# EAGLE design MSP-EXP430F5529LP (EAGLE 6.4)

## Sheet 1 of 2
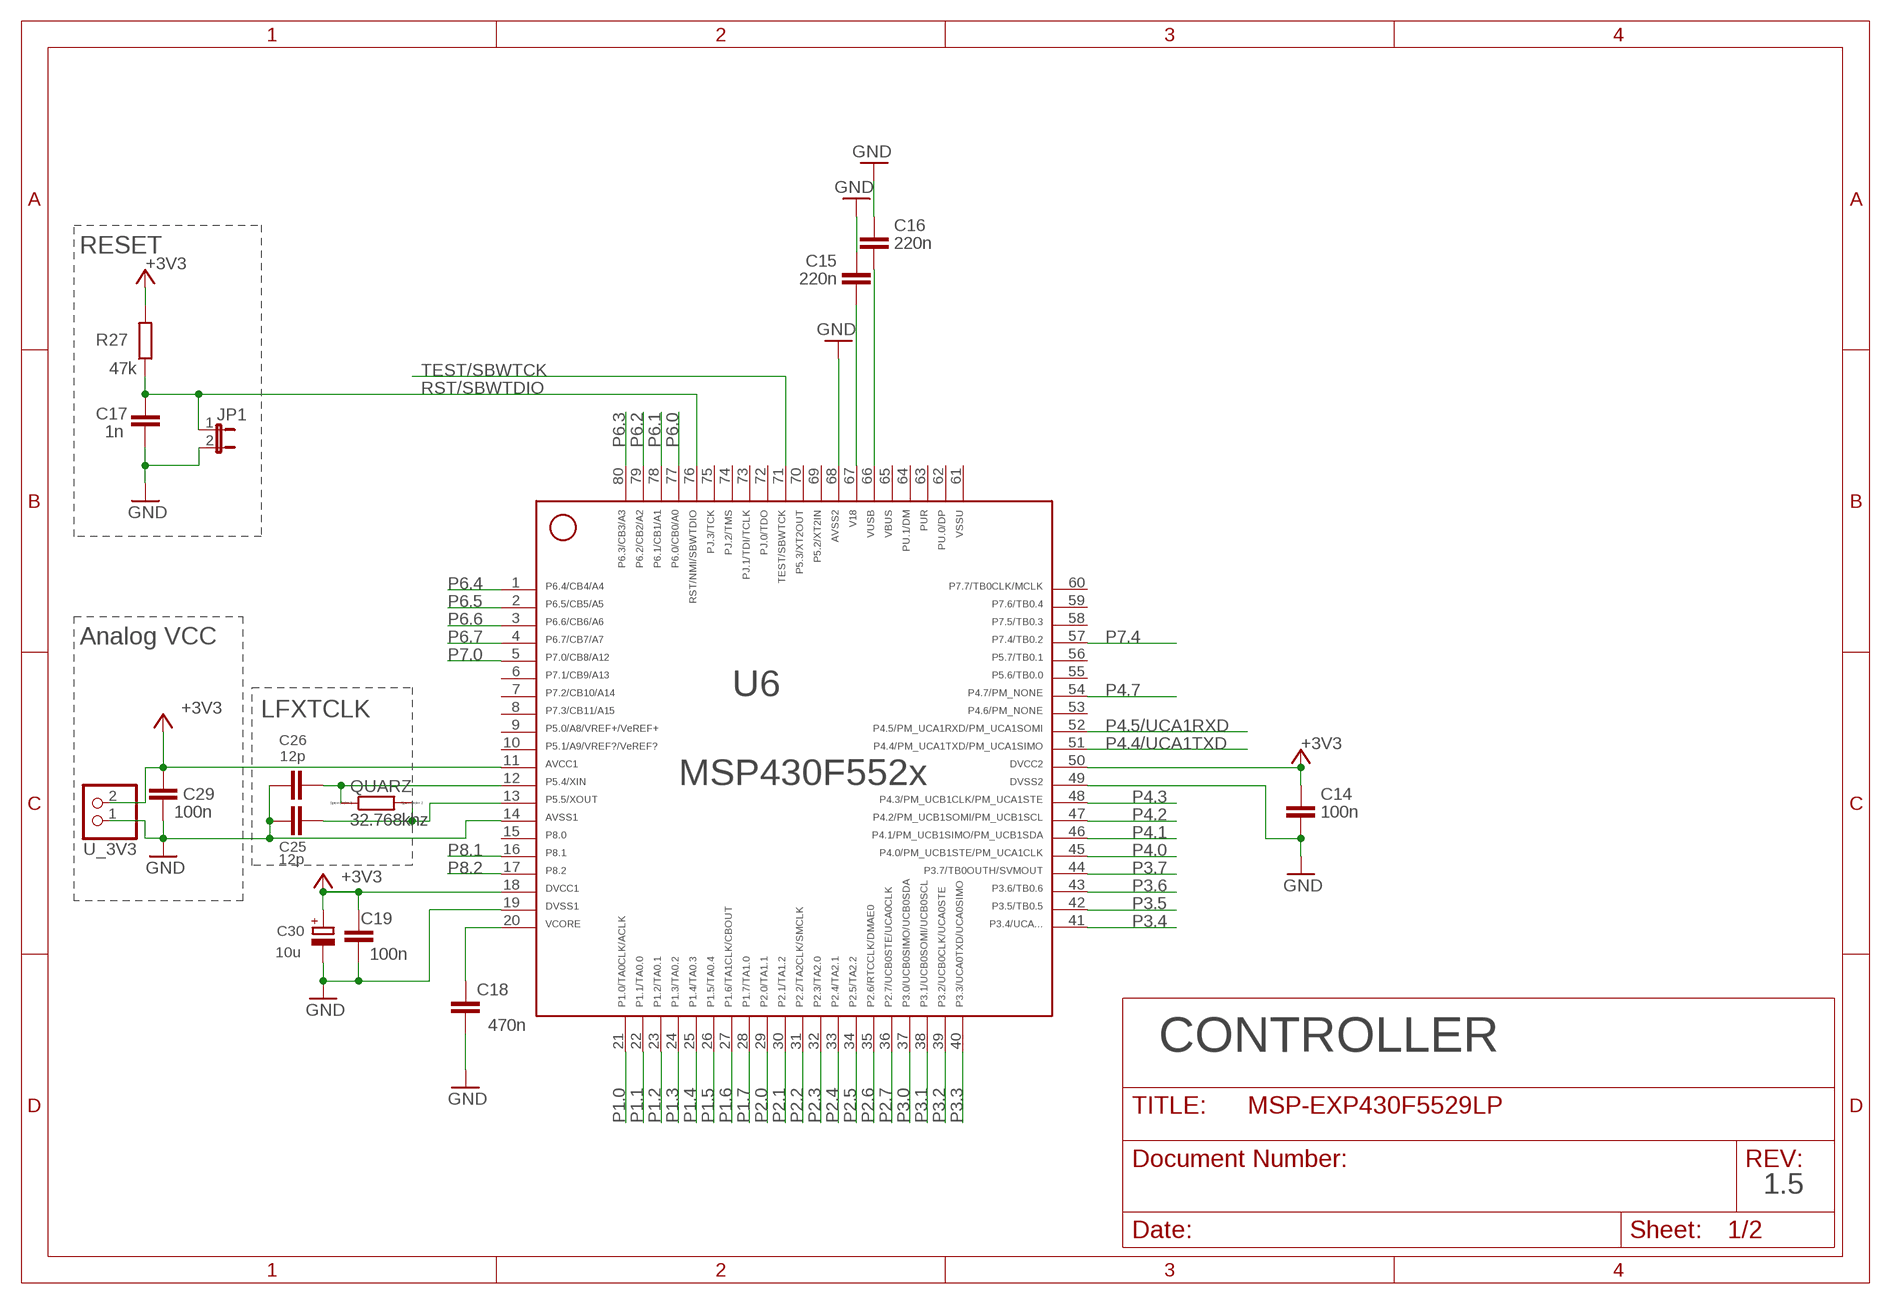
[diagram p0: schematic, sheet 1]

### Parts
C14  100n  C-EUC0402  [C0402]
C15  220n  C-EUC0805  [C0805]
C16  220n  C-EUC0805  [C0805]
C17  1n  C-EUC0805  [C0805]
C18  470n  C-EUC0805  [C0805]
C19  100n  C-EUC0603  [C0603]
C25  12p  C-EUC0805  [C0805]
C26  12p  C-EUC0805  [C0805]
C29  100n  C-EUC0603  [C0603]
C30  10u  CPOL-EUA/3216-18R  [A/3216-18R]
JP1  JP1E  [JP1]
QUARZ  32.768khz  RR1206  [R1206]
R27  47k  R-EU_R0603  [R0603]
U6  MSP430F5529IPNR  F552X---PN80  [PN80]
U_3V3  PINHD-1X2  [1X02]

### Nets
+3V3 [Power]: C14.1 C19.2 C29.1 C30.+ R27.2 U6.11 U6.18 U6.50 U_3V3.2 ; also sheet 2
GND [Ground]: C14.2 C15.2 C16.2 C17.2 C18.1 C19.1 C25.1 C26.1 C29.2 C30.- JP1.2 U6.14 U6.19 U6.49 U6.68 U_3V3.1 ; also sheet 2
P1.0: U6.21 ; also sheet 2
P1.1: U6.22
P1.2: U6.23 ; also sheet 2
P1.3: U6.24 ; also sheet 2
P1.4: U6.25 ; also sheet 2
P1.5: U6.26 ; also sheet 2
P1.6: U6.27 ; also sheet 2
P1.7: U6.28
P2.0: U6.29
P2.1: U6.30
P2.2: U6.31
P2.3: U6.32
P2.4: U6.33
P2.5: U6.34
P2.6: U6.35 ; also sheet 2
P2.7: U6.36
P3.0: U6.37 ; also sheet 2
P3.1: U6.38
P3.2: U6.39 ; also sheet 2
P3.3: U6.40 ; also sheet 2
P3.4: U6.41
P3.5: U6.42 ; also sheet 2
P3.6: U6.43 ; also sheet 2
P3.7: U6.44
P4.0: U6.45
P4.1: U6.46 ; also sheet 2
P4.2: U6.47
P4.3: U6.48 ; also sheet 2
P4.4/UCA1TXD: U6.51 ; also sheet 2
P4.5/UCA1RXD: U6.52 ; also sheet 2
P4.7: U6.54 ; also sheet 2
P5.4/XIN: C26.2 QUARZ.1 U6.12
P5.5/XOUT: C25.2 QUARZ.2 U6.13
P6.0: U6.77 ; also sheet 2
P6.1: U6.78 ; also sheet 2
P6.2: U6.79 ; also sheet 2
P6.3: U6.80 ; also sheet 2
P6.4: U6.1
P6.5: U6.2
P6.6: U6.3
P6.7: U6.4
P7.0: U6.5
P7.4: U6.57 ; also sheet 2
P8.1: U6.16 ; also sheet 2
P8.2: U6.17
RST/SBWTDIO: C17.1 JP1.1 R27.1 U6.76 ; also sheet 2
TARGET_VUSB [Power]: C16.1 U6.66
TEST/SBWTCK: U6.71 ; also sheet 2
V18 [Power]: C15.1 U6.67
VCORE [Power]: C18.2 U6.20
Unconnected: U6.6 U6.7 U6.8 U6.9 U6.10 U6.15 U6.53 U6.55 U6.56 U6.58 U6.59 U6.60 U6.62 U6.63 U6.64 U6.69 U6.70 U6.72 U6.73 U6.74 U6.75

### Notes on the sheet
- RESET
- Analog VCC
- LFXTCLK
- CONTROLLER
- 1.5

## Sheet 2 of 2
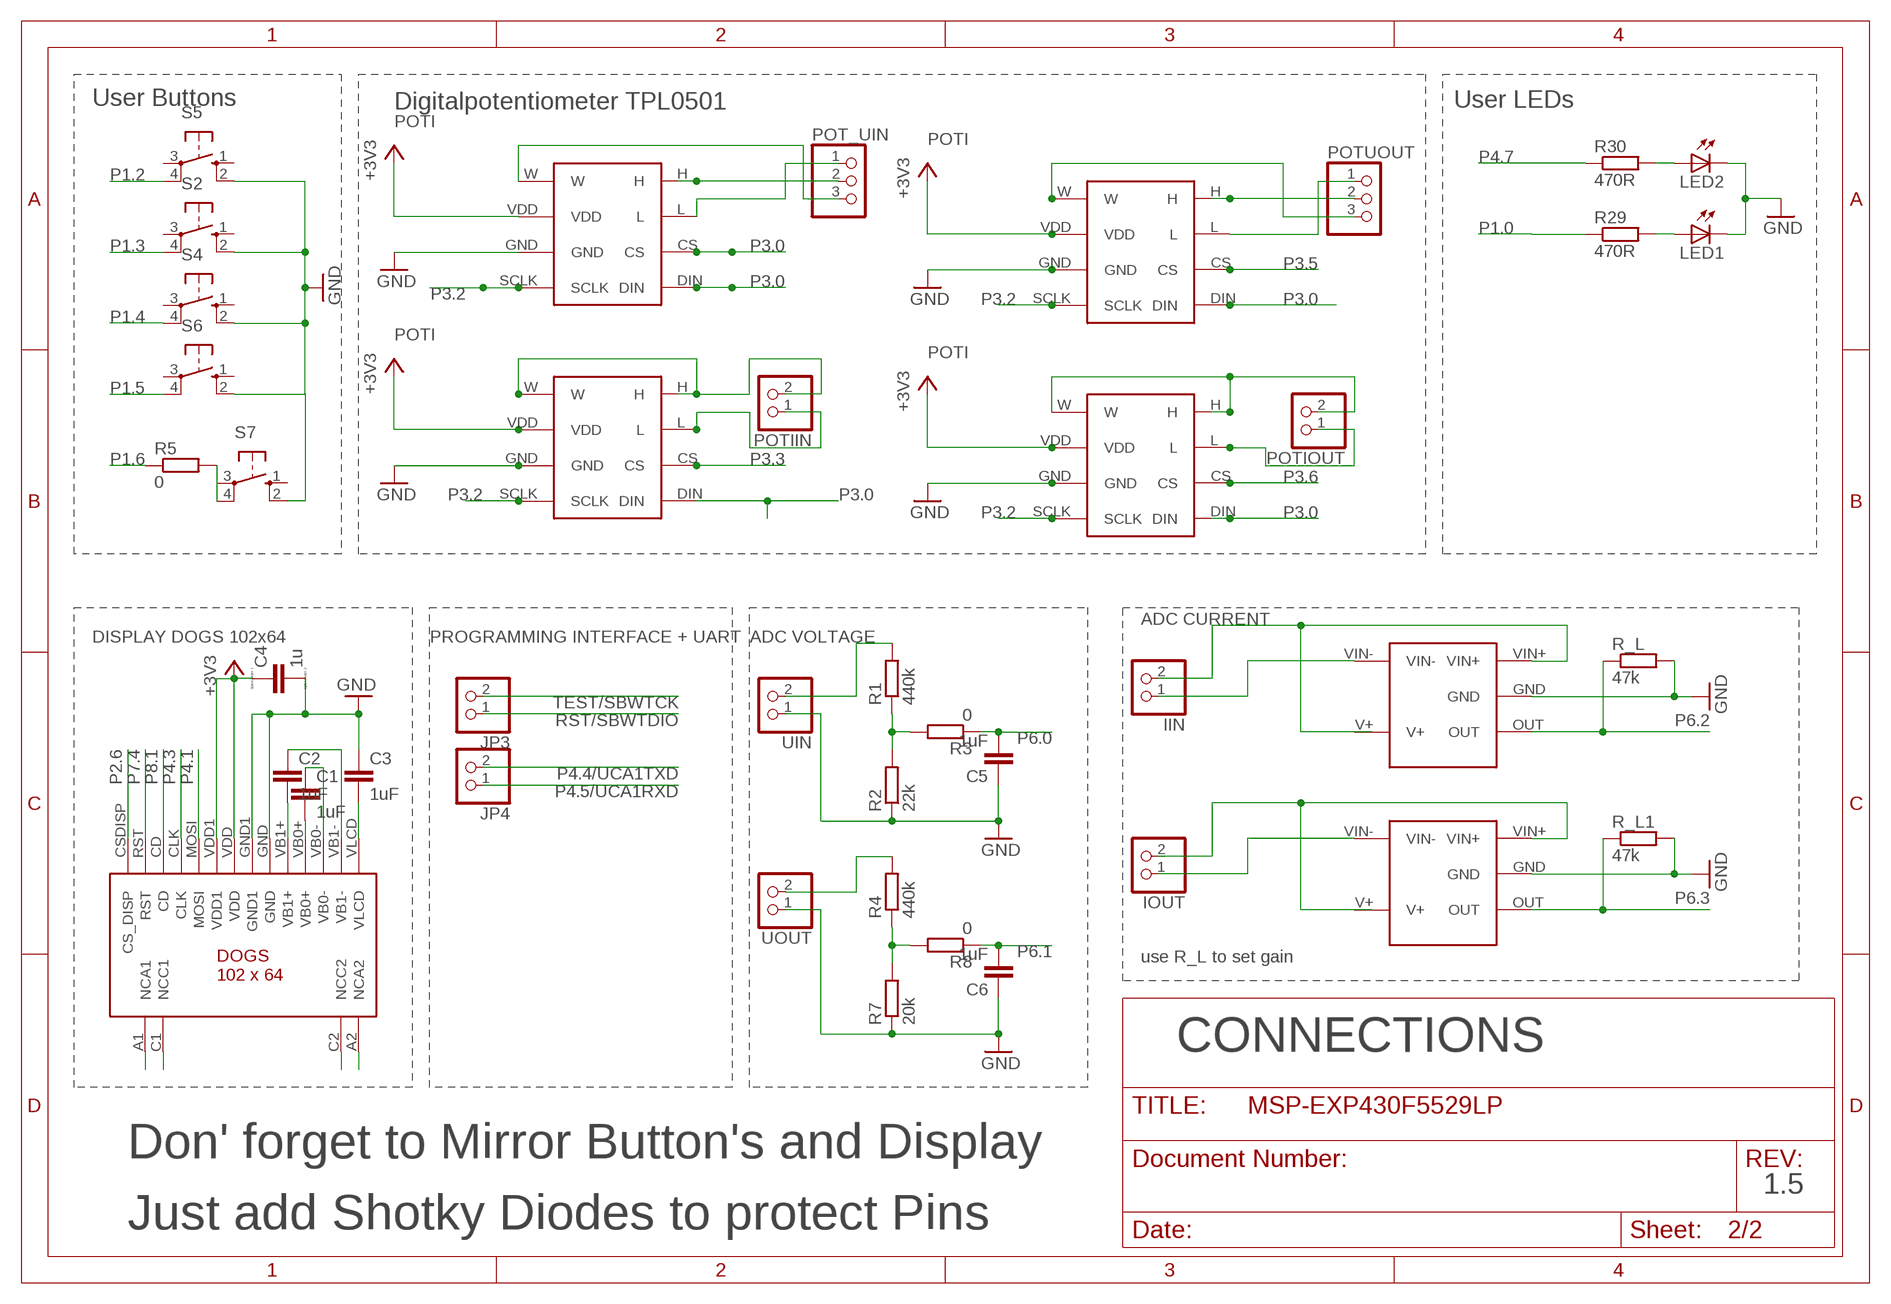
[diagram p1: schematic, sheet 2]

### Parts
C1  1uF  C-EUC0805  [C0805]
C2  1uF  C-EUC0805  [C0805]
C3  1uF  C-EUC0805  [C0805]
C4  1u  C  [C0805]
C5  1uF  C-EUC0805  [C0805]
C6  1uF  C-EUC0805  [C0805]
IIN  PINHD-1X2  [1X02]
IOUT  PINHD-1X2  [1X02]
JP3  PINHD-1X2  [1X02]
JP4  PINHD-1X2  [1X02]
LED1  LEDCHIP-LED0805  [CHIP-LED0805]
LED2  LEDCHIPLED_0603  [CHIPLED_0603]
POT_UIN  PINHD-1X3  [1X03]
POTIIN  PINHD-1X2  [1X02]
POTIOUT  PINHD-1X2  [1X02]
POTUOUT  PINHD-1X3  [1X03]
R1  440k  R-EU_MELF0204W  [MINI_MELF-0204W]
R2  22k  R-EU_R0805  [R0805]
R3  0  R-EU_R0805  [R0805]
R4  440k  R-EU_R0805  [R0805]
R5  0  R-EU_R0805  [R0805]
R7  20k  R-EU_R0805  [R0805]
R8  0  R-EU_R0805  [R0805]
R29  470R  R-EU_R0805  [R0805]
R30  470R  R-EU_R0603  [R0603]
R_L  47k  R-EU_M0805  [M0805]
R_L1  47k  R-EU_M0805  [M0805]
S2  10-XX  [B3F-10XX]
S4  10-XX  [B3F-10XX]
S5  10-XX  [B3F-10XX]
S6  10-XX  [B3F-10XX]
S7  10-XX  [B3F-10XX]
U$1  INA138  [SOT23-5]
U$2  INA138  [SOT23-5]
U$4  TPL0501  [SOT23-8L]
U$6  TPL0501  [SOT23-8L]
U$7  TPL0501  [SOT23-8L]
U$8  TPL0501  [SOT23-8L]
U$9  DOGS102  [1X14]
UIN  PINHD-1X2  [1X02]
UOUT  PINHD-1X2  [1X02]

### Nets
+3V3 [Power]: C4.1 U$4.VDD U$6.VDD U$7.VDD U$8.VDD U$9.VDD U$9.VDD1 ; also sheet 1
GND [Ground]: C3.1 C4.2 C5.1 C6.1 LED1.C LED2.C R2.1 R7.1 R_L1.2 R_L.2 S2.2(S1) S4.2(S1) S5.2(S1) S6.2(S1) S7.2(S1) U$1.GND U$2.GND U$4.GND U$6.GND U$7.GND U$8.GND U$9.GND U$9.GND1 UIN.1 UOUT.1 ; also sheet 1
N$1: POT_UIN.2 U$4.H
N$2: POTIIN.1 U$6.L
N$3: POT_UIN.1 U$4.L
N$4: POT_UIN.3 U$4.W
N$5: POTUOUT.3 U$8.W
N$6: IIN.2 U$1.VIN+
N$7: C2.2 U$9.VB1+
N$8: POTIOUT.1 U$7.L
N$9: R1.1 R2.2 R3.2
N$12: POTIIN.2 U$6.H U$6.W
N$13: POTUOUT.2 U$8.H
N$14: POTUOUT.1 U$8.L
N$15: R5.2 S7.4(P1)
N$16: C1.2 U$9.VB0+
N$17: C1.1 U$9.VB0-
N$18: C2.1 U$9.VB1-
N$19: C3.2 U$9.VLCD
N$22: U$9.A1(NCA1)
N$23: U$9.C1(NCC1)
N$24: IIN.1 U$1.VIN-
N$26: R1.2 UIN.2
N$28: U$9.C2(NCC2)
N$30: IOUT.2 U$2.VIN+
N$32: LED1.A R29.2
N$34: IOUT.1 U$2.VIN-
N$35: LED2.A R30.2
N$36: U$9.A2(NCA2)
N$37: R4.1 R7.2 R8.2
N$39: R4.2 UOUT.2
N$44: POTIOUT.2 U$7.H U$7.W
P1.0: R29.1 ; also sheet 1
P1.2: S5.4(P1) ; also sheet 1
P1.3: S2.4(P1) ; also sheet 1
P1.4: S4.4(P1) ; also sheet 1
P1.5: S6.4(P1) ; also sheet 1
P1.6: R5.1 ; also sheet 1
P2.6: U$9.CSDISP(CS_DISP) ; also sheet 1
P3.0: U$4.CS U$4.DIN U$6.DIN U$7.DIN U$8.DIN ; also sheet 1
P3.2: U$4.SCLK U$6.SCLK U$7.SCLK U$8.SCLK ; also sheet 1
P3.3: U$6.CS ; also sheet 1
P3.5: U$8.CS ; also sheet 1
P3.6: U$7.CS ; also sheet 1
P4.1: U$9.MOSI ; also sheet 1
P4.3: U$9.CLK ; also sheet 1
P4.4/UCA1TXD: JP4.2 ; also sheet 1
P4.5/UCA1RXD: JP4.1 ; also sheet 1
P4.7: R30.1 ; also sheet 1
P6.0: C5.2 R3.1 ; also sheet 1
P6.1: C6.2 R8.1 ; also sheet 1
P6.2: R_L.1 U$1.OUT ; also sheet 1
P6.3: R_L1.1 U$2.OUT ; also sheet 1
P7.4: U$9.RST ; also sheet 1
P8.1: U$9.CD ; also sheet 1
RST/SBWTDIO: JP3.1 ; also sheet 1
TEST/SBWTCK: JP3.2 ; also sheet 1
Unconnected: S2.1(S) S2.3(P) S4.1(S) S4.3(P) S5.1(S) S5.3(P) S6.1(S) S6.3(P) S7.1(S) S7.3(P) U$1.V+ U$2.V+

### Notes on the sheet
- User Buttons | Digitalpotentiometer TPL0501 | User LEDs
- POTI
- POTI
- POTI
- POTI
- ADC CURRENT
- DISPLAY DOGS 102x64 | PROGRAMMING INTERFACE + UART | ADC VOLTAGE
- use R_L to set gain
- CONNECTIONS
- Don' forget to Mirror Button's and Display
- 1.5
- Just add Shotky Diodes to protect Pins

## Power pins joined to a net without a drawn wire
61: U6.61
65: U6.65

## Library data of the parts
C1-C3 C5 C6 C14-C19 C25 C26 C29 = rcl:C-EU: CAPACITOR, European symbol
C4 = eagle-ltspice:C: CAPACITOR, European symbol; SPICEMODEL: NONE; SPICEPREFIX: C
C30 = rcl:CPOL-EU: POLARIZED CAPACITOR, European symbol
IIN IOUT JP3 JP4 POTIIN POTIOUT U_3V3 UIN UOUT = pinhead:PINHD-1X2: PIN HEADER
JP1 = jumper:JP1E: JUMPER
LED1 LED2 = led:LED: LED
POT_UIN POTUOUT = pinhead:PINHD-1X3: PIN HEADER
QUARZ = eagle-ltspice:R: RESISTOR, European symbol; SPICEMODEL: NONE; SPICEPREFIX: R
R1-R5 R7 R8 R27 R29 R30 R_L R_L1 = rcl:R-EU_: RESISTOR, European symbol
S2 S4-S7 = switch-omron:10-XX: OMRON SWITCH; MPN: B3F-1000; OC_FARNELL: 176432; OC_NEWARK: 36M3542
U6 = TI_MSP430_v16_intern:F552X---PN80: ***MSP430F552X***PN80 http://www.ti.com/lit/gpn/msp430f5529 Rev1.0 06/2010 For F552X where X is 1,5,7,9
U$1 U$2 = current_shunt:INA138
U$4 U$6-U$8 = tpl0501:TPL0501
U$9 = dogs_102x64:DOGS102

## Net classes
0 Default: width 0.203 mm, drill 0.305 mm, clearance 0.152 mm
1 Ground: width 0.203 mm, drill 0.305 mm, clearance 0.152 mm to class 0, clearance 0.152 mm
2 Power: width 0.203 mm, drill 0.305 mm, clearance 0.152 mm to class 0, clearance 0.152 mm to class 1, clearance 0.152 mm

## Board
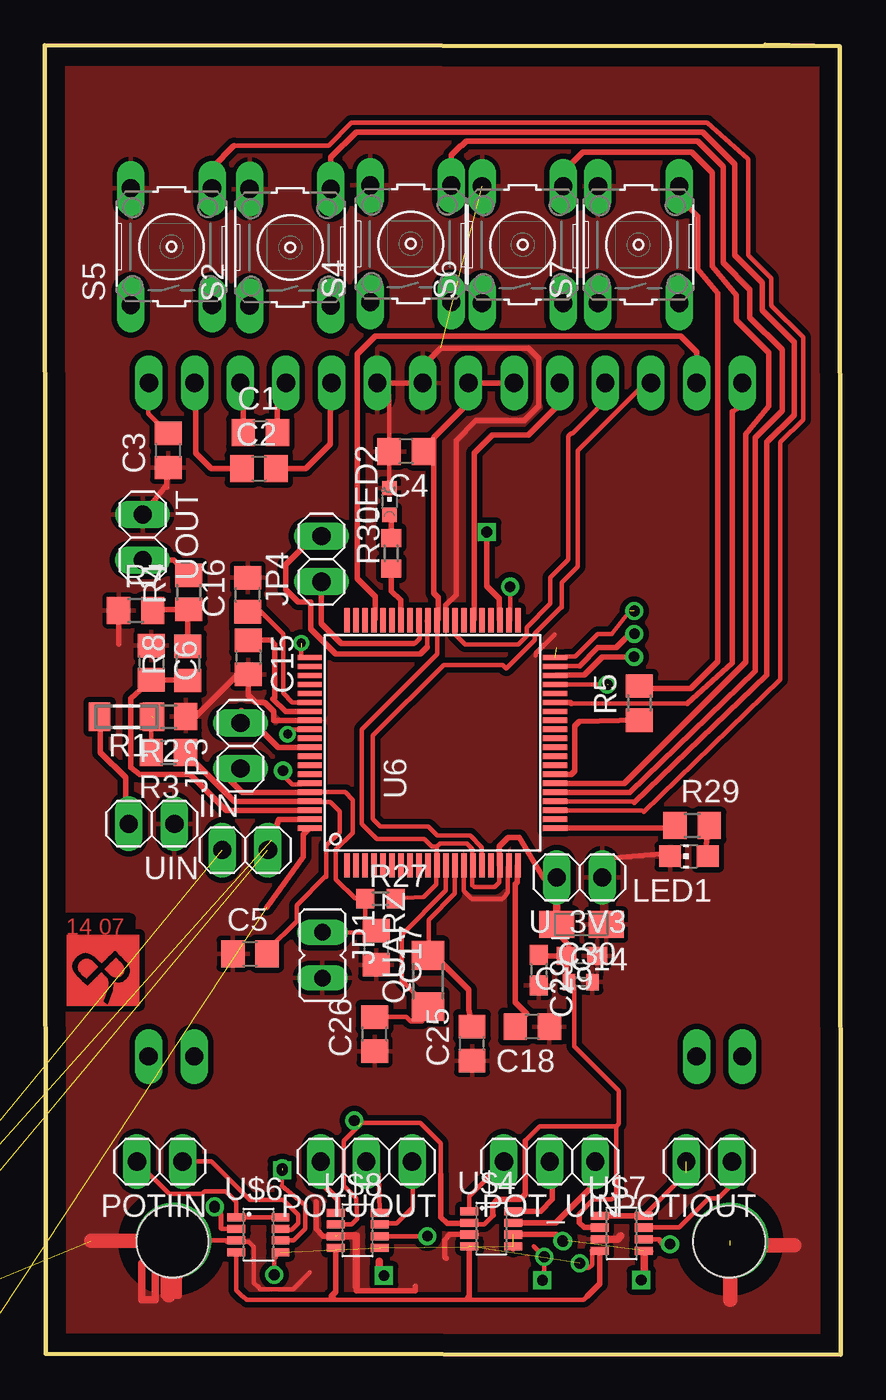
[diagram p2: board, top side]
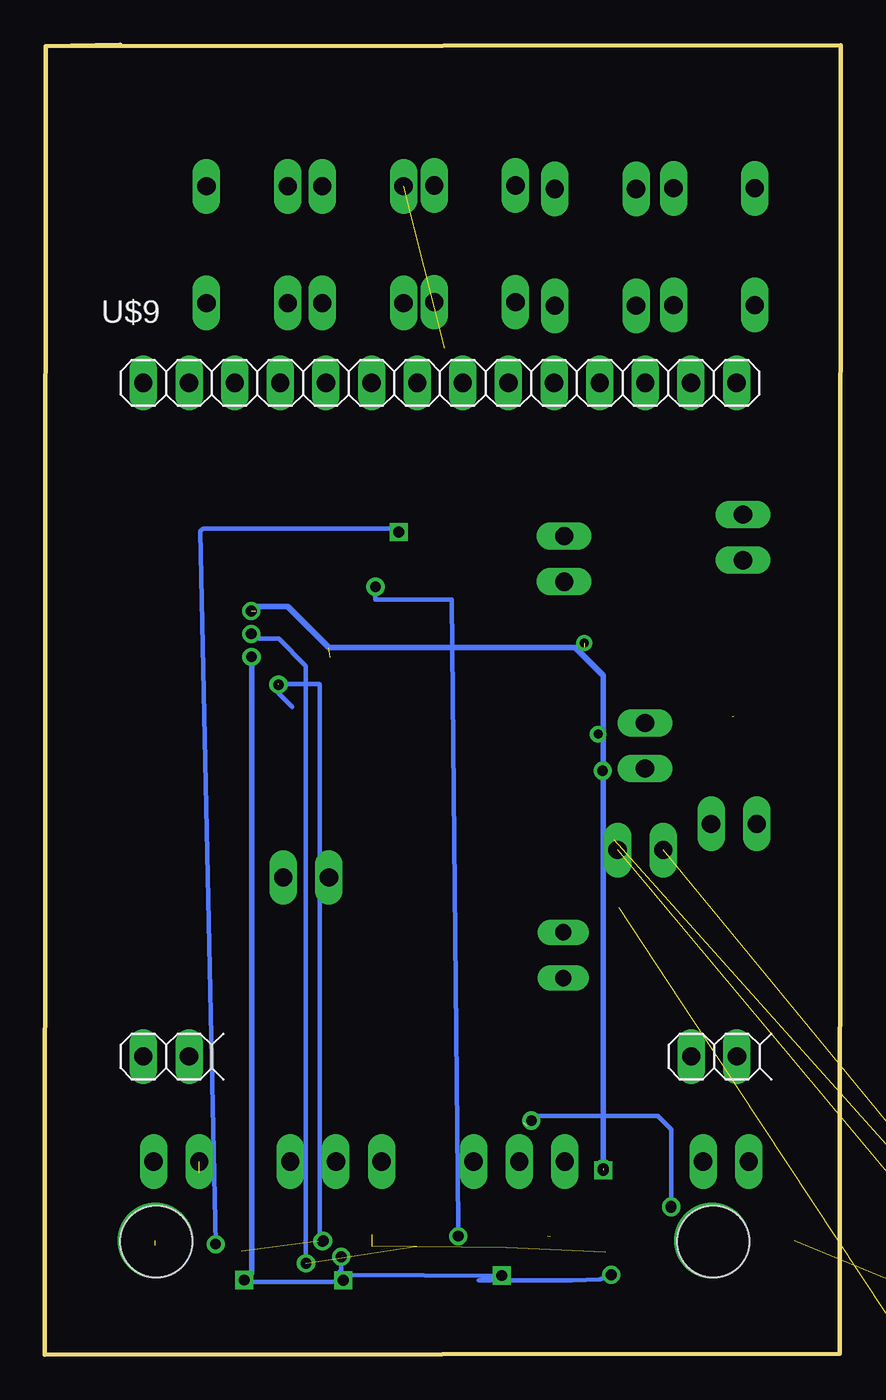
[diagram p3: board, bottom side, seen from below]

Size 44.29 x 72.92 mm. Coordinates in mm from the lower left corner, seen from the top.
Outline: 40.09,72.92 44.25,72.84
Outline: 44.25,72.84 44.29,0 0.04,0.05 0,72.89 44.25,72.84
Copper layers (1*16): Top 0.035mm / dielectric 1.5mm / Bottom 0.035mm
Design rules "default": minimum track width 10mil, minimum drill 24mil, track to track 8mil, track to pad 8mil, pad to pad 8mil, via to via 8mil, smd to smd 8mil, copper to edge 40mil, drill to drill 8mil, minimum pad ring 10mil, minimum via ring 8mil, stop-mask expansion 4mil, vias tented up to drill 0mil, thermal gap 10mil
Holes 4 mm at 7.09,6.3 38.09,6.3

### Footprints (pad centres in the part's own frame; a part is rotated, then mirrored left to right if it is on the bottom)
C0805 = smd 1.3 x 1.5: 1 -0.95,0; 2 0.95,0
C0402 = smd 0.7 x 0.9: 1 -0.65,0; 2 0.65,0
C0603 = smd 1.1 x 1: 1 -0.85,0; 2 0.85,0
A/3216-18R = smd 1.95 x 1.5: + 1.375,0; - -1.375,0
1X02 = drill 1.016 long: 1 -1.27,0; 2 1.27,0
JP1 = drill 0.914 long: 1 0,-1.27; 2 0,1.27
CHIP-LED0805 = smd 1.2 x 1.2: A 0,-1.05; C 0,1.05
CHIPLED_0603 = smd 0.8 x 0.8: A 0,-0.75; C 0,0.75
1X03 = drill 1.016 long: 1 -2.54,0; 2 0,0; 3 2.54,0
R1206 = smd 1.6 x 1.803: 1 -1.422,0; 2 1.422,0
MINI_MELF-0204W = smd 1.2 x 1.6: 1 -1.5,0; 2 1.5,0
R0805 = smd 1.3 x 1.5: 1 -0.95,0; 2 0.95,0
R0603 = smd 1 x 1.1: 1 -0.85,0; 2 0.85,0
M0805 = smd 1.3 x 1.6: 1 -0.95,0; 2 0.95,0
B3F-10XX = drill 1.016 long: 1 -3.251,2.261; 2 3.251,2.261; 3 -3.251,-2.261; 4 3.251,-2.261
PN80 = smd 1.35 x 0.3: 1 -6.825,4.75; 2 -6.825,4.25; 3 -6.825,3.75; 4 -6.825,3.25; 5 -6.825,2.75; 6 -6.825,2.25; 7 -6.825,1.75; 8 -6.825,1.25; 9 -6.825,0.75; 10 -6.825,0.25; 11 -6.825,-0.25; 12 -6.825,-0.75; 13 -6.825,-1.25; 14 -6.825,-1.75; 15 -6.825,-2.25; 16 -6.825,-2.75; 17 -6.825,-3.25; 18 -6.825,-3.75; 19 -6.825,-4.25; 20 -6.825,-4.75; 41 6.825,-4.75; 42 6.825,-4.25; 43 6.825,-3.75; 44 6.825,-3.25; 45 6.825,-2.75; 46 6.825,-2.25; 47 6.825,-1.75; 48 6.825,-1.25; 49 6.825,-0.75; 50 6.825,-0.25; 51 6.825,0.25; 52 6.825,0.75; 53 6.825,1.25; 54 6.825,1.75; 55 6.825,2.25; 56 6.825,2.75; 57 6.825,3.25; 58 6.825,3.75; 59 6.825,4.25; 60 6.825,4.75 | smd 0.3 x 1.35: 21 -4.75,-6.825; 22 -4.25,-6.825; 23 -3.75,-6.825; 24 -3.25,-6.825; 25 -2.75,-6.825; 26 -2.25,-6.825; 27 -1.75,-6.825; 28 -1.25,-6.825; 29 -0.75,-6.825; 30 -0.25,-6.825; 31 0.25,-6.825; 32 0.75,-6.825; 33 1.25,-6.825; 34 1.75,-6.825; 35 2.25,-6.825; 36 2.75,-6.825; 37 3.25,-6.825; 38 3.75,-6.825; 39 4.25,-6.825; 40 4.75,-6.825; 61 4.75,6.825; 62 4.25,6.825; 63 3.75,6.825; 64 3.25,6.825; 65 2.75,6.825; 66 2.25,6.825; 67 1.75,6.825; 68 1.25,6.825; 69 0.75,6.825; 70 0.25,6.825; 71 -0.25,6.825; 72 -0.75,6.825; 73 -1.25,6.825; 74 -1.75,6.825; 75 -2.25,6.825; 76 -2.75,6.825; 77 -3.25,6.825; 78 -3.75,6.825; 79 -4.25,6.825; 80 -4.75,6.825
SOT23-5 = smd 0.6 x 1.2: GND 0,-1.306; OUT -0.95,-1.306; V+ -0.95,1.306; VIN+ 0.95,-1.306; VIN- 0.95,1.306
SOT23-8L = smd 0.45 x 1: CS 0.325,1.225; DIN 0.975,1.225; GND 0.325,-1.225; H -0.975,1.225; L -0.325,1.225; SCLK 0.975,-1.225; VDD -0.325,-1.225; W -0.975,-1.225
1X14 = drill 1.016 long: A1 3.08,1.59; A2 36.12,1.59; C1 5.62,1.59; C2 33.58,1.59; CD 8.16,39.09; CLK 10.7,39.09; CSDISP 3.08,39.09; GND 23.4,39.09; GND1 20.86,39.09; MOSI 13.24,39.09; RST 5.62,39.09; VB0+ 28.48,39.09; VB0- 31.02,39.09; VB1+ 25.94,39.09; VB1- 33.56,39.09; VDD 18.32,39.09; VDD1 15.78,39.09; VLCD 36.1,39.09

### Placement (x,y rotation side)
C1  11.99,51.33 0 top
C2  11.91,49.33 0 top
C3  6.86,50.34 90 top
C4  20.11,50.29 180 top
C5  11.41,22.32 0 top
C6  5.92,38.52 270 top
C14  29.83,20.74 0 top
C15  11.31,38.83 270 top
C16  11.29,42.31 90 top
C17  18.44,22.66 270 top
C18  27.13,18.26 180 top
C19  29.89,22.2 180 top
C25  23.77,17.32 90 top
C26  18.35,17.85 90 top
C29  27.48,21.4 270 top
C30  29.86,23.95 180 top
IIN  11.15,28.09 0 top
IOUT  not placed on the board
JP1  15.44,22.24 180 top
JP3  10.89,33.9 90 top
JP4  15.39,44.3 90 top
LED1  35.84,27.74 90 top
LED2  19.17,47.5 0 top
POT_UIN  28.09,10.75 180 top
POTIIN  6.39,10.75 180 top
POTIOUT  36.97,10.75 180 top
POTUOUT  17.89,10.75 180 top
QUARZ  21.32,20.8 90 top
R1  4.54,35.51 180 top
R2  6.89,35.52 180 top
R3  6.87,33.52 180 top
R4  8.01,42.44 90 top
R5  33.09,36.28 90 top
R7  5.05,41.43 0 top
R8  7.96,38.48 90 top
R27  18.69,25.39 0 top
R29  36.03,29.46 0 top
R30  19.27,44.62 90 top
R_L  not placed on the board
R_L1  not placed on the board
S2  13.65,61.65 90 top
S4  20.36,61.85 90 top
S5  7.04,61.69 90 top
S6  26.59,61.8 90 top
S7  33.04,61.8 90 top
U6  21.57,34.06 90 top
U$1  not placed on the board
U$2  not placed on the board
U$4  24.85,7.01 270 top
U$6  11.89,6.68 270 top
U$7  32.1,6.75 270 top
U$8  17.4,6.92 270 top
U$9  41.89,15.01 0 bottom
U_3V3  29.76,26.57 180 top
UIN  5.94,29.55 180 top
UOUT  5.44,45.5 270 top

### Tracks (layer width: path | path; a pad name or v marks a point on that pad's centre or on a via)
+3V3  (via drill 0.6)  (1 unrouted)
  Top 0.254: U$8.VDD 17.09,7.24 17.39,7.55 17.34,8.7 16.64,9.4 16.64,11.9 17.64,12.9 20.89,12.9 22.04,11.75 22.04,10.05 | 23.04,7.3 23.59,7.3 | 26.74,11.9 27.54,12.7 31.79,12.7 | 24.94,7.75 24.44,7.25 23.71,7.25 U$4.VDD | C14.1 29.46,20.46 29.46,17.17 31.94,14.69 31.94,12.85 31.79,12.7 | R27.2 21.09,25.49 21.79,26.19 21.79,27.2 U6.11 21.82,28.28 | U6.50 21.84,40.87 21.84,39.01 17.62,34.8 17.62,29.54 18.46,28.7 21.13,28.7 21.54,28.28 21.82,28.28 | 25.29,27.27 25.29,26.29 25.04,26.03 23.89,26.03 23.79,26.14 23.79,28.17 23.49,28.47 22.01,28.47 21.82,28.28 | v9.44,8.25 9.8,7.9 9.8,7.03 9.83,7 U$6.VDD 9.88,7 9.82,7.06 9.82,7.82 v9.44,8.2 | 29.74,7.8 29.74,7.85 30.52,8.63 31.54,8.63 31.79,8.89 31.79,12.7
  Top 0.305: U$9.VDD1 U$9.VDD 23.57,52.99 21.63,51.05 21.63,50.54 | U_3V3.2 27.76,26.52 26.39,28.8 25.79,28.8 25.29,28.3 25.29,27.27 U6.18 | C30.+ 28.48,23.5 29.16,22.82 29.16,22.32 C19.2 | C19.2 29.04,20.88 C14.1 | C19.2 27.53,22.2 C29.1 | U$7.VDD 30.02,7.07 29.74,7.35 29.74,7.8 | 22.04,10.05 22.04,7.65 22.39,7.3 23.59,7.3 U$4.VDD | 21.63,50.54 21.63,42.42 21.89,42.16 21.89,40.95 U6.50 | 26.74,11.9 26.74,8.92 26.46,8.63 25.19,8.63 24.94,8.38 24.94,7.76 24.94,7.75 | C4.1 21.38,50.29 21.63,50.54
  Top 0.406: U_3V3.2 28.48,26.52 C30.+
  Bottom 0.254: v9.44,8.2 9.44,12.55 10.18,13.28 16.88,13.28 17.45,12.71
GND  (via drill 3.2 pad 1.02)  (7 unrouted)
  Top 0.254: LED2.C 19.17,53.42 U$9.GND | 27.32,38.94 27.32,39.06 | 27.32,39.06 27.81,39.55 | 27.32,39.06 27.35,39.06 28.39,40.1 | U6.14 23.32,25.82 23.77,25.37 25.44,25.37 25.67,25.6 25.67,25.65 25.75,25.73 25.75,27.16 U6.19 | U$6.GND 9.25,6.36 9.06,6.17 9.06,5.71 7.92,4.57 | 10.13,6.27 11.35,6.27 11.63,5.99 11.63,4.01 11.93,3.71 11.93,3.68 11.98,3.63 13.81,3.63 14.75,4.57
  Top 0.305: U$9.GND U$9.GND1 21.03,55.04 22.04,56.05 26.89,56.05 27.49,55.45 27.49,52.8 26.69,52 23.99,52 22.89,50.9 22.89,42.3 22.32,41.73 U6.49 | R7.1 4.1,39.57 | 5.84,39.39 C6.1 | UOUT.1 6.72,48.37 6.79,48.3 6.79,49.25 6.94,49.4 6.99,49.4 7.04,49.35 6.89,49.35 6.79,49.45 | U$8.GND 15.5,6.59 15.09,7 15.09,8.5 | U$4.GND 22.53,6.68 22.24,6.4 22.24,5.45 22.34,5.35 22.34,5.4 | 31.47,26.86 31.47,27.51 31.36,27.62 34.63,27.9 LED1.C | R2.1 8.39,35.52 10.71,37.84 | C15.2 11.31,36.74 11.73,36.32 12.24,36.32 12.74,35.81 12.74,35.3 14.74,35.3 U6.68 | 17.32,3.81 17.32,3.55 20.62,3.55 20.62,3.81
  Top 0.406: 5.63,5.08 5.38,5.08 5.38,3.05 6.14,3.05 6.14,4.57 6.65,4.57 6.65,3.3 6.9,3.3 7.41,3.3 7.41,4.32 7.66,4.57 7.92,4.57 | U$7.GND 31.87,6.42 32.05,6.6 | 16.3,6.6 17.32,6.6 17.32,3.81
  Top 0.813: 38.14,6.09 41.7,6.09 | 38.14,5.84 38.14,3.05 | 2.58,6.35 6.9,6.35 6.9,3.3
  other vias: 38.14,6.35
  pour Top (isolate 0.305): -7.81,72.7 46.79,73.15 46.04,-0.05 -7.31,-0.5
  pour Top: 16.05,38.35 20.36,38.35 17.06,35.05 17.06,32 16.05,32
N$1
  Top 0.305: U$4.H 27.59,7.98 28.24,8.63 28.24,10.6 POT_UIN.2
N$2
  Top 0.254: POTIIN.1 9.26,10.75 11.4,8.61 13.28,8.61 14.09,7.8 14.09,7.31 13.74,6.96 13.16,6.96 U$6.L
N$3
  Top 0.305: U$4.L 28.43,7.33 31.09,10 31.09,10.29 POT_UIN.1
N$4
  Top 0.254: 25.43,10.75 POT_UIN.3 23.63,8.82 U$4.W
N$5
  Top 0.305: POTUOUT.3 15.35,9.58 16.3,8.63 16.3,8.02 U$8.W
N$6  (1 unrouted)
N$7
  Top 0.305: C2.2 14.52,49.33 15.89,50.7 15.89,54.04 U$9.VB1+
N$8
  Top 0.254: U$7.L 35.31,7.07 36.95,8.71 37.48,8.71 38.35,9.57 38.35,10.64 POTIOUT.1
N$9  (1 unrouted)
  Top 0.254: R3.2 5.92,35.5 R2.2
N$12
  Top 0.254: U$6.H U$6.W 10.66,8.51 10.08,9.09 8.9,9.09 8.74,8.94 6.93,8.94 POTIIN.2
N$13
  Top 0.254: U$8.H 18.58,10.06 POTUOUT.2
N$14
  Top 0.254: POTUOUT.1 20.48,8.19 19.59,7.3 18.68,7.3 U$8.L
N$15
  Top 0.305: S7.4 35.3,64.44 36.34,63.4 36.34,60.45 37.44,59.1 37.44,54.05 37.44,53.8 37.44,38.6 35.94,37.1 33.14,37.1 R5.2
N$16
  Top 0.305: C1.2 12.94,53.63 U$9.VB0+
N$17
  Top 0.305: C1.1 11.04,53.93 U$9.VB0-
N$18
  Top 0.305: C2.1 9.26,49.33 8.39,50.2 8.39,54.04 U$9.VB1-
N$19
  Top 0.254: 5.76,54.07 5.76,52.39 C3.2
  Top 0.305: 5.76,54.07 U$9.VLCD
N$20  (via drill 0.6)
  other vias: 31.29,37.3
N$21  (via drill 0.6)
  other vias: 25.89,42.75
N$24  (1 unrouted)
N$26
  Top 0.305: UIN.2 4.49,30.17 4.49,32.13 3.09,33.53 3.09,35.47 R1.2
N$27  (via drill 0.6)
  other vias: 13.25,32.51
N$29  (via drill 0.6)
  other vias: 17.21,13.03
N$30  (1 unrouted)
N$31
  Top 0.254: 14.27,31.75 13.76,31.75 13.25,32.26
N$32
  Top 0.305: R29.2 36.72,27.91 LED1.A
N$33  (via drill 3.2 pad 1.02)
  other vias: 7.16,6.35
N$34  (1 unrouted)
N$35
  Top 0.305: R30.2 19.27,46.65 LED2.A
N$37
  Top 0.305: R8.2 7.96,41.44 R4.1 6.06,41.49 R7.2
N$38  (via drill 0.5)  (1 unrouted)
  Top 0.254: 14.27,38.86 14.27,39.37
  other vias: 14.27,39.62
N$39
  Top 0.305: UOUT.2 7.17,44.23 R4.2
N$42  (via drill 0.5)
  other vias: 13.51,34.54
N$43
  Top 0.254: 14.52,34.8 13.51,34.8
N$44  (1 unrouted)
  Top 0.254: 35.7,10.1 U$7.H
  Top 0.305: U$7.W U$7.H
P1.0
  Top 0.305: U6.21 34.67,29.31 R29.1
P1.2
  Top 0.254: S5.4 9.3,66.15 10.46,67.31 15.79,67.31 17.06,68.58 36.87,68.58 39.16,66.55 39.16,61.21 40.43,59.94 40.43,58.42 42.21,56.64 42.21,52.07 40.94,50.8 40.94,37.59 33.32,30.22 33.23,30.31 U6.23
  Top 0.305: S5.4 9.3,66.06 10.54,67.3
P1.3
  Top 0.254: U6.24 32.73,30.81 32.81,30.73
  Top 0.305: S2.4 15.91,66.67 17.32,68.07 36.62,68.07 38.4,66.29 38.4,61.21 39.92,59.69 39.92,58.16 41.7,56.39 41.7,52.32 40.18,50.8 40.18,37.84 32.81,30.73
P1.4
  Top 0.305: S4.4 22.62,66.78 23.14,67.3 23.19,67.3 23.44,67.55 36.34,67.55 37.74,66.15 37.74,60.8 39.24,59.3 39.24,57.75 41.05,55.95 41.05,52.55 39.55,51.05 39.55,38.05 32.54,31.3 28.41,31.3 U6.25
P1.5
  Top 0.305: S6.4 28.85,65.86 29.94,66.95 35.99,66.95 37.14,65.8 37.14,60.6 38.49,59 38.49,57.6 40.29,55.8 40.29,52.8 39,51.25 39,38.55 32.24,31.8 28.41,31.8 U6.26
P1.6
  Top 0.305: R5.1 29.74,35.25 29.49,35 29.49,32.5 29.29,32.3 28.41,32.3 U6.27
P2.6
  Top 0.254: 29.29,36.25 35.74,36.25
  Top 0.305: U$9.CSDISP 38.81,52.82 38.25,52.51 38.25,38.5 35.74,36.25 | 29.29,36.25 29.24,36.3 28.41,36.3 U6.35
P3.0  (via drill 0.6)  (5 unrouted)
  Top 0.254: v28.81,6.33 v28.84,6.3 | U6.37 29.59,37.31 31.34,37.3 | U$4.DIN 26.08,5.83
  Top 0.305: U$4.CS 28.46,6.68 v28.81,6.33
  Bottom 0.254: 29.09,6.33 v28.81,6.33 29,6.53 29,37.31 29.04,37.35 31.29,37.35 31.29,36.83 30.52,36.07
P3.1  (via drill 0.6)
  Top 0.254: 27.21,6.04 v27.79,5.45 27.79,4.75 v27.69,4.14 | 33.29,4.25 v33.19,4.15 | v12.77,4.45 12.77,5.41
  Top 0.305: v32.79,38.85 31.02,38.85 30.02,37.84 28.43,37.84 U6.38 | 12.77,5.41 12.82,5.41
  Top 0.406: 18.62,5.2 18.62,4.65 v18.87,4.4 | 33.66,5.75 33.35,5.75 33.35,4.31 v33.19,4.15
  Bottom 0.254: v12.77,4.45 13.38,4.19 14.94,4.15 20.14,4.15 v18.87,4.4 27.49,4.45 v27.69,4.14 28.29,4.05 32.79,4.05 | v27.79,5.45 27.79,4.7 28.04,4.45 | v33.19,4.15 32.79,4.05 | 33.24,4.5 32.79,4.05
  Bottom 0.305: v32.79,38.85 32.79,4.55 v33.19,4.15
P3.2  (via drill 0.6)  (1 unrouted)
  Top 0.254: 29.76,38.35 28.44,38.35 U6.39 | U$6.SCLK 10.66,3.58 10.99,3.25 11.02,3.25 11.22,3.05 16.05,3.05 | 16.05,3.05 29.99,3.05 30.38,3.44 | 15.94,3.25 15.94,3.15 16.05,3.05 | 30.46,5.78 30.46,5.01 30.27,4.82 30.02,4.82 v29.76,5.08
  Top 0.305: U$8.SCLK 16.19,5.93 16.19,3.5 15.94,3.25 16.04,3.15 | U$4.SCLK 23.63,3.23 23.54,3.15 | 30.18,3.23 30.38,3.44 30.88,3.93 U$7.SCLK 30.46,5.78 | v32.81,40.13 32.56,40.13 31.79,39.37 30.78,39.37 29.76,38.35
  Bottom 0.254: v29.76,5.08 29.76,38.35 31.29,39.88 32.56,39.88 v32.81,40.13
P3.3  (via drill 0.6)  (3 unrouted)
  Top 0.2: v13.21,10.26 13.21,9.42 13.19,9.4
  Top 0.254: U$6.CS 13.85,6.36 14.49,7 14.49,8.3 13.19,9.4 | 29,38.86 29.51,38.86 30.78,40.13 31.54,40.13 32.56,41.4
  Bottom 0.305: v13.21,10.26 13.21,37.8 14.78,39.37 28.49,39.37 30.78,41.65 32.56,41.65 v32.81,41.4
  other vias: 13.21,10.36
P3.5  (via drill 0.6)  (1 unrouted)
  Top 0.254: U$8.CS v21.29,6.59 | U6.42 25.89,40.88 25.89,42.55
  Bottom 0.254: v21.29,6.59 21.29,7.2 21.64,42.05 25.89,42.05 25.89,42.55
P3.6  (via drill 0.6)
  Top 0.254: 34.24,6.3 34.12,6.42 U$7.CS 34.22,6.42
  Top 0.305: v24.59,45.8 24.59,42.8 25.29,42.1 25.29,40.91 U6.43 | v34.79,6.15 34.39,6.15 34.24,6.3
  Bottom 0.254: v34.79,6.15 35.64,45.85 35.49,46 24.79,46 v24.59,45.8
P4.1
  Top 0.305: U$9.MOSI 28.65,52.96 26.89,51.2 24.89,51.2 23.89,50.2 23.89,40.95 U6.46
P4.3
  Top 0.254: U6.48 22.82,40.11 23.39,39.55 26.36,39.55 26.82,40 26.82,40.49 28.14,41.81 28.14,43.28 29.13,44.27 29.13,51.13 29.28,51.28 29.36,51.28 31.11,53.03 31.11,54.02 U$9.CLK
P4.4/UCA1TXD
  Top 0.254: 21.29,39.4 21.29,40.85
  Top 0.305: JP4.2 14.96,45.57 13.39,44 13.39,42.6 14.09,41.9 14.79,41.9 14.79,40.4 16.19,39 20.89,39 21.29,39.4 | 21.29,40.85 U6.51
P4.5/UCA1RXD
  Top 0.254: 20.49,39.6 20.6,39.6 20.87,39.88 20.87,40.83 U6.52
  Top 0.305: JP4.1 15.39,40.7 16.49,39.6 20.49,39.6
P4.7
  Top 0.305: R30.1 19.27,42.52 19.79,42 19.79,40.91 U6.54
P5.4/XIN
  Top 0.254: C26.2 20.11,18.8 20.36,18.54 21.01,18.54 QUARZ.1 19.86,20.85 19.86,23.37 22.32,25.83 U6.12
  Top 0.305: QUARZ.1 21.71,19.38
P5.5/XOUT
  Top 0.254: U6.13 22.82,25.67 21.36,24.2 21.36,22.7 QUARZ.2
  Top 0.305: 22.83,27.23 U6.13 | QUARZ.2 21.83,22.06 23.59,20.3 23.59,19.21 C25.2
P6.0
  Top 0.254: C5.2 12.36,22.53 12.41,22.53 14.01,24.13 14.01,25.02 15.67,26.67 | 15.67,26.59 15.67,26.67 | 15.67,26.67 15.67,28.34 16.4,29.08 16.4,30.25 15.87,30.78 14.77,30.78 U6.77
  Top 0.305: U6.77 10.53,30.81 R3.1
P6.1
  Top 0.305: U6.78 10.08,30.31 8.09,32.3 5.29,32.3 4.79,32.7 4.79,36.54 C6.2 7.92,37.57 R8.1
P6.2  (2 unrouted)
  Top 0.305: 12.62,28.66 13,29.81 U6.79
P6.3  (2 unrouted)
  Top 0.305: 12.35,24.89 14.39,27.7 14.39,28.96 U6.80
P7.4
  Top 0.305: U$9.RST 36.27,55.82 35.39,56.7 18.39,56.7 17.39,55.7 17.39,43.2 18.39,42.2 18.39,40.95 U6.57
P8.1
  Top 0.254: U$9.CD 33.42,54.1 29.66,50.34 29.66,43.89 28.77,43 28.77,41.6 28.72,41.6 27.27,40.15 27.27,39.8 25.67,38.2 25.47,38.4 22.19,38.4 18.26,34.47 18.26,29.82 18.66,29.41 21.33,29.41 21.84,28.9 23.67,28.9 24.33,28.24 U6.16
RST/SBWTDIO
  Top 0.254: JP1.1 17.71,23.51 | 17.71,23.51 18.1,23.11 18.13,23.11 18.18,23.16 18.18,23.36 C17.1 | U6.76 16.71,31.32 17.14,30.88 17.14,29.06 16.2,28.12 16.2,26.46 17.27,25.39 R27.1 17.84,23.64 17.71,23.51
  Top 0.305: JP3.1 10.09,32.2 10.99,31.3 14.74,31.3 U6.76
TARGET_VUSB
  Top 0.254: C16.1 12.02,41.36 13.25,40.13 13.25,36.83 13.76,36.32 14.74,36.32 U6.66
TEST/SBWTCK
  Top 0.305: JP3.2 10.92,35.87 12.99,33.8 14.74,33.8 U6.71
V18
  Top 0.305: U6.67 14.74,35.8 13.39,35.8 12.69,36.5 12.79,36.6 12.79,39.55 12.56,39.78 C15.1
VCORE
  Top 0.305: C18.2 26.81,18.98 26.19,19.6 26.19,26.2 26.29,26.3 26.29,27.21 U6.20
(copper drawn outside any net)
  shapes: Top area x420

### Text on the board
Top: 14 07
